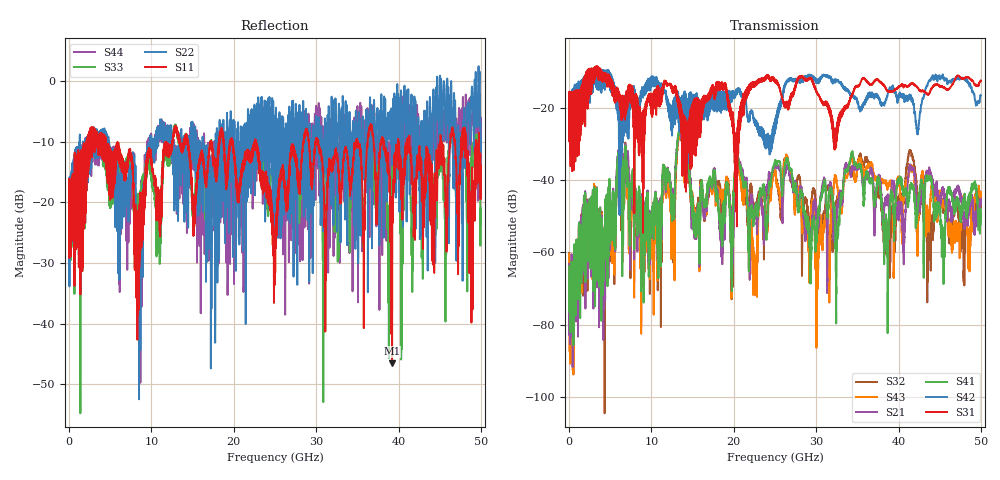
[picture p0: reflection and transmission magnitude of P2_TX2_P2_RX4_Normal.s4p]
!Keysight Technologies,N5225B,MY57041031,A.13.20.10
!Date: Friday, May 31, 2019 11:32:30
!Correction: S11(Full 4 Port(1,2,3,4))
!S12(Full 4 Port(1,2,3,4))
!S13(Full 4 Port(1,2,3,4))
!S14(Full 4 Port(1,2,3,4))
!S21(Full 4 Port(1,2,3,4))
!S22(Full 4 Port(1,2,3,4))
!S23(Full 4 Port(1,2,3,4))
!S24(Full 4 Port(1,2,3,4))
!S31(Full 4 Port(1,2,3,4))
!S32(Full 4 Port(1,2,3,4))
!S33(Full 4 Port(1,2,3,4))
!S34(Full 4 Port(1,2,3,4))
!S41(Full 4 Port(1,2,3,4))
!S42(Full 4 Port(1,2,3,4))
!S43(Full 4 Port(1,2,3,4))
!S44(Full 4 Port(1,2,3,4))
!S4P File: Measurements: <S11,S12,S13,S14>,
!<S21,S22,S23,S24>,
!<S31,S32,S33,S34>,
!<S41,S42,S43,S44>:
# Hz S  dB  R 50.0
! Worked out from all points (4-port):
!   5000 points, 10 MHz to 50 GHz, reference 50 ohm
!   strongest paths, dB at 10 MHz, 12.51 GHz, 25.01 GHz, 37.51 GHz, 50 GHz:
!     S31: -19.3, -14.9, -13.0, -12.4, -12.6
!     S42: -19.7, -27.8, -23.9, -17.0, -16.7
!     S41: -63.9, -45.4, -34.6, -39.1, -51.4
!     S21: -63.2, -42.6, -35.6, -39.7, -45.8
!     S43: -60.4, -55.5, -37.5, -39.9, -44.4
!     S32: -60.2, -49.4, -37.6, -42.6, -45.1
!   lowest |S11| = -46.5 dB at 39.22 GHz (marker M1), VSWR 1.01, Z = 50 + j0.473 ohm
!   |S11| at or under -10 dB: 4.481 GHz to 11.72 GHz (7.238 GHz wide, 89.4 % of centre); 22.72 GHz to 28.43 GHz (5.704 GHz wide, 22.3 % of centre); 30.26 GHz to 34.82 GHz (4.56 GHz wide, 14 % of centre)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
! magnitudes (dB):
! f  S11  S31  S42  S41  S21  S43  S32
! 10 MHz  -19.1  -19.3  -19.7  -63.9  -63.2  -60.4  -60.2
! 13.55 GHz  -10.4  -20.2  -20.7  -25.9  -26.9  -26.6  -27.4
! 22.58 GHz  -9.9  -13.9  -24.1  -48.3  -48.6  -66.1  -46.4
! 26.37 GHz  -21.0  -19.3  -13.0  -34.2  -36.5  -33.0  -33.5
! 30.14 GHz  -9.8  -16.1  -13.1  -52.7  -51.1  -63.3  -50.7
! 39.22 GHz  -46.5  -15.7  -14.4  -43.7  -41.1  -42.6  -50.3
! 50 GHz  -14.0  -12.6  -16.7  -51.4  -45.8  -44.4  -45.1
